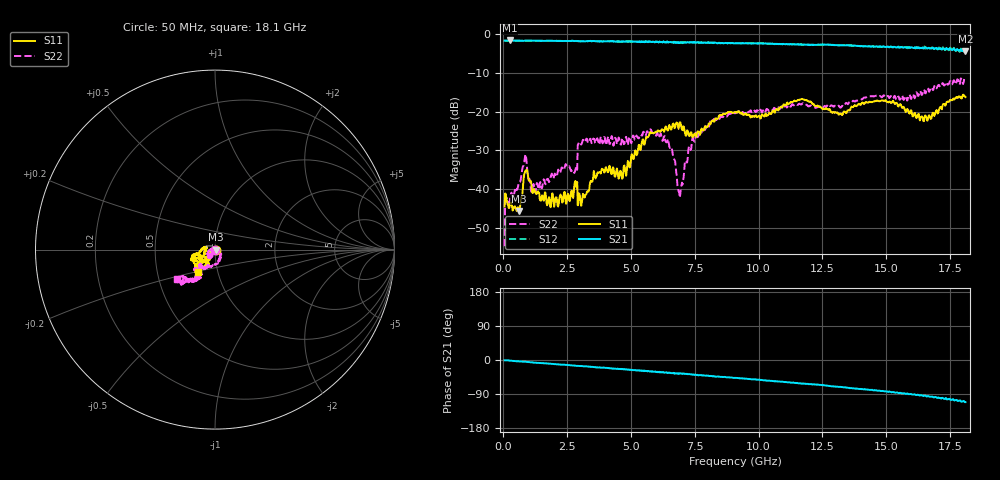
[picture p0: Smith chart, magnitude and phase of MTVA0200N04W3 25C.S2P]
! Network Analyzer HP8720D.06.14 Serial No. US36140669
! 17 Jan 2005  12:43:10
! Frequency  S11  S21  S12  S22
# HZ  S  DB R 50
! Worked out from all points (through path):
!   801 points, 50 MHz to 18.1 GHz, reference 50 ohm
!   highest |S21| = -1.56 dB at 253.1 MHz (marker M1); lowest = -4.4 dB at 18.1 GHz (marker M2)
!   group delay of S21, straight-line fit = 16 ps
!   lowest |S11| = -45.7 dB at 614.1 MHz (marker M3), VSWR 1.01, Z = 50.5 - j0.118 ohm
!   |S11| at or under -10 dB: start of sweep to end of sweep
!   |S22| runs from -54.8 to -11.1 dB; largest |S21 - S12| = 0.033
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5e7  -44.51 -35.4  -1.58 -0.7  -1.61 -0.9  -54.75 -23.0
1.628125e8  -43.83 -20.7  -1.60 -0.8  -1.62 -1.2  -42.96 -34.0
2.530625e8  -44.31 -20.0  -1.56 -1.6  -1.57 -2.0  -42.89 -43.5
6.140625e8  -45.67 -12.9  -1.60 -3.7  -1.61 -3.7  -38.17 -67.4
8.848125e8  -35.31 -32.8  -1.59 -4.7  -1.59 -5.0  -31.36 -124.5
1.04275e9  -37.84 -60.3  -1.58 -5.7  -1.59 -6.0  -37.81 -145.7
1.3135e9  -41.14 -67.7  -1.63 -7.3  -1.64 -7.5  -38.42 -127.5
2.080625e9  -42.10 -79.1  -1.67 -11.2  -1.65 -11.5  -36.83 -136.3
2.802625e9  -38.13 -86.3  -1.72 -14.7  -1.67 -15.3  -35.50 -151.7
3.073375e9  -43.39 -140.1  -1.73 -16.1  -1.71 -16.4  -28.21 -115.2
3.614875e9  -37.23 -100.9  -1.74 -18.9  -1.73 -19.4  -28.16 -124.3
4.607625e9  -35.44 -128.6  -1.87 -23.4  -1.88 -24.1  -28.50 -124.9
6.074188e9  -24.85 -131.5  -2.02 -32.2  -2.03 -32.4  -26.37 -142.5
6.525438e9  -23.78 -126.7  -2.00 -33.8  -2.06 -33.7  -29.38 -161.8
6.931562e9  -22.70 -149.9  -2.11 -35.9  -2.21 -36.2  -41.39 67.8
7.473062e9  -25.80 168.9  -1.95 -38.6  -2.00 -39.3  -27.59 -48.2
9.075e9  -20.09 -154.9  -2.28 -47.0  -2.28 -47.4  -20.38 -107.0
1.209838e10  -17.79 -151.6  -2.64 -64.3  -2.66 -64.5  -18.63 -135.7
1.320394e10  -20.48 -147.7  -2.80 -71.0  -2.78 -71.6  -18.92 -130.4
1.509919e10  -17.47 -134.4  -3.31 -83.8  -3.24 -84.8  -16.21 -136.8
1.654319e10  -21.01 -129.3  -3.43 -94.6  -3.66 -96.2  -15.25 -120.9
1.81e10  -16.20 -127.7  -4.38 -111.2  -4.18 -112.4  -11.46 -142.3
